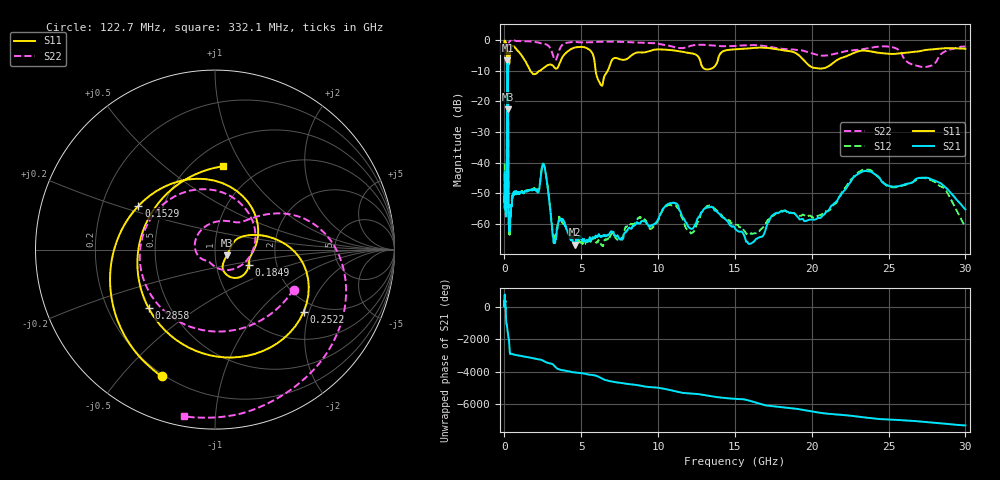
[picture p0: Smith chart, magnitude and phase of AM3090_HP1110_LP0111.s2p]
! Date/Time: Thu, Feb 28, 2019 2:09 PM
! Network Analyzer: Agilent Technologies E8364B Rev: A.07.50.67
! Sweep from 0.010 to 30.000 GHz, 1601 Points, Sweep Type: LOG
! Power Supply: 5.022 V, 0.002 A
# Hz S DB R 50
!freq MagS11 AngS11 MagS21 AngS21 MagS12 AngS12 MagS22 AngS22
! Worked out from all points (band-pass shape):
!   1601 points, 10 MHz to 30 GHz, reference 50 ohm
!   highest |S21| = -6.68 dB at 195.4 MHz (marker M1); lowest = -66.8 dB at 4.571 GHz (marker M2)
!   |S21| within 3 dB of the highest: 172.9 MHz to 225.3 MHz (52.35 MHz wide, 26.3 % of centre)
!   lowest |S11| = -22.7 dB at 213.8 MHz (marker M3), VSWR 1.16, Z = 57 - j3.54 ohm
!   |S11| at or under -10 dB: 165.3 MHz to 235.6 MHz (70.28 MHz wide, 35.1 % of centre); 1.677 GHz to 2.353 GHz (676.3 MHz wide, 33.6 % of centre); 5.931 GHz to 6.721 GHz (790.5 MHz wide, 12.5 % of centre)
!   |S22| runs from -22.4 to -0.2 dB; largest |S21 - S12| = 0.016
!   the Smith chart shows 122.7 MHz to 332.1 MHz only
!   S11 on the Smith chart (normalised r, x): 122.7 MHz: 0.19, -0.65; 152.9 MHz: 0.36, +0.23; 184.9 MHz: 1.43, -0.25; 252.2 MHz: 1.69, -1.84; 285.8 MHz: 0.38, -0.33; 332.1 MHz: 0.70, +0.83
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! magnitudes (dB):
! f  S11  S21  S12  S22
! 10 MHz  -0.3  -43.0  -40.3  -0.6
! 38.04 MHz  -0.3  -52.5  -51.2  -1.3
! 122.7 MHz  -2.3  -53.0  -52.1  -6.2
! 144.7 MHz  -4.5  -48.5  -47.8  -7.4
! 152.9 MHz  -6.2  -35.3  -35.1  -8.6
! 184.9 MHz  -13.7  -7.1  -7.1  -21.9
! 195.4 MHz  -13.7  -6.7  -6.7  -19.2
! 213.8 MHz  -22.7  -7.5  -7.4  -15.7
! 252.2 MHz  -4.4  -35.2  -35.8  -2.7
! 285.8 MHz  -6.1  -60.1  -58.9  -1.0
! 332.1 MHz  -6.6  -60.6  -60.7  -0.5
! 550.5 MHz  -2.0  -50.9  -50.7  -0.3
! 2.084 GHz  -10.9  -49.2  -48.3  -0.7
! 2.558 GHz  -9.1  -40.6  -40.6  -1.3
! 3.22 GHz  -8.8  -66.0  -64.1  -6.1
! 4.571 GHz  -2.5  -66.8  -65.1  -0.7
! 6.234 GHz  -14.3  -64.1  -66.3  -0.6
! 7.926 GHz  -6.3  -62.6  -60.9  -0.7
! 10.86 GHz  -3.3  -53.3  -53.9  -2.1
! 16.29 GHz  -2.6  -65.5  -63.1  -1.7
! 23.48 GHz  -3.5  -42.8  -42.3  -2.9
! 30 GHz  -2.9  -55.3  -61.0  -2.2
